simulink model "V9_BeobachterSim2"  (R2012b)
settings: Solver=ode4  SolverMode=SingleTasking  StartTime=0.0  StopTime=5  FixedStep=0.001  RelTol=1e-3
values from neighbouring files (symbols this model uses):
  A = [-2 1    [V9_1_Beobachterdesign.m]    (also in V9_2_Beobachterdesign.m; V9_3_Beobachterdesign.m)
  B = [1; 1]    [V9_1_Beobachterdesign.m]    (also in V9_2_Beobachterdesign.m = [0; 1]; V9_3_Beobachterdesign.m = [0; 1])
  C = [1 0]    [V9_1_Beobachterdesign.m]    (also in V9_2_Beobachterdesign.m; V9_3_Beobachterdesign.m; LinProb.m = LinProb(A.GetSize()))
  G = place(A',C',poles)    [V9_1_Beobachterdesign.m]    (also in V9_2_Beobachterdesign.m; V2_6_UTFDiskretizierung.m = tf(1,[1 1]))
  K = place(A,B,pc)    [V9_2_Beobachterdesign.m]    (also in V9_3_Beobachterdesign.m = place(Ad,Bd,pcd); kalman1.m = sys(2)/(sigma*sigma); kalman2.m = sys(2)/(sigma*sigma); kalman3.m = sys(2)/(r2))

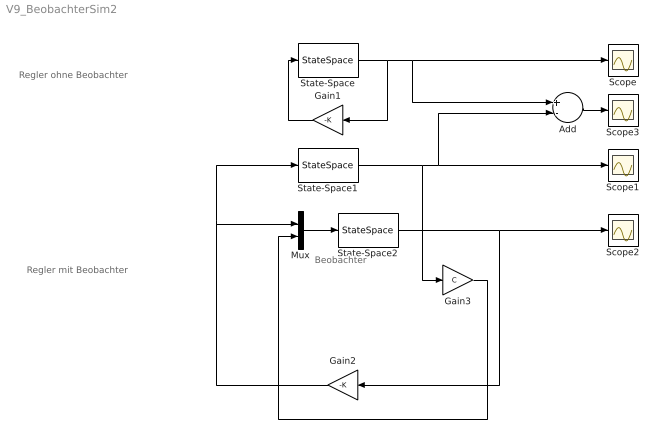
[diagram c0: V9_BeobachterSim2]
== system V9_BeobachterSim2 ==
  note: Beobachter
  note: Regler mit Beobachter
  note: Regler ohne Beobachter
  Add : Sum  Inputs=+-
  Gain1 : Gain  Gain=-K  Multiplication=Matrix(K*u)
  Gain2 : Gain  Gain=-K  Multiplication=Matrix(K*u)
  Gain3 : Gain  Gain=C  Multiplication=Matrix(K*u)
  Mux : Mux  Inputs=2
  Scope{,1..3} (4 alike) : Scope
  State-Space : StateSpace  A=A  B=B  C=eye(2)  D=[0; 0]  X0=[2; 1]
  State-Space1 : StateSpace  A=A  B=B  C=eye(2)  D=[0; 0]  X0=[2; 1]
  State-Space2 : StateSpace  A=A-G'*C  B=[B G']  C=eye(2)  D=zeros(2,2)  X0=[0; 0]
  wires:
  Mux/1 -> State-Space2/1
  Gain3/1 -> Mux/2
  State-Space/1 -> Gain1/1, Scope/1, Add/1
  State-Space1/1 -> Gain3/1, Add/2, Scope1/1
  Add/1 -> Scope3/1
  State-Space2/1 -> Scope2/1, Gain2/1
  Gain1/1 -> State-Space/1
  Gain2/1 -> Mux/1, State-Space1/1
